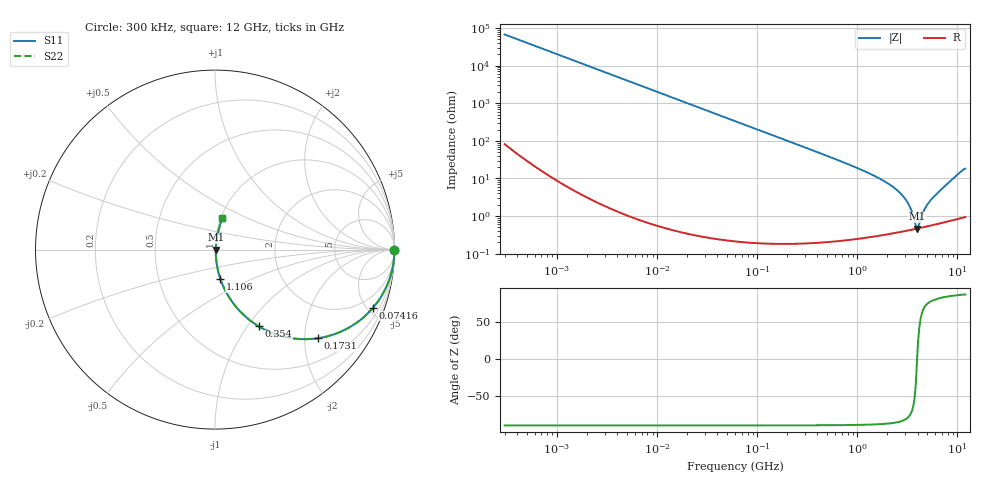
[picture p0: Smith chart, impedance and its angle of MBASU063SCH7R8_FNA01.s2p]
! MBASU063SCH7R8_FNA01  S-PARAMETER MODEL  ( General Type )
! Model Generated by TAIYO YUDEN Corporation (http://www.ty-top.com)
! Version 1.0
! TAIYO YUDEN Control No. 130801
! Copyright(c) 2013 TAIYO YUDEN CO.,LTD. All Rights Reserved.
! Product Description (link to TY-COMPAS)
! https://ds.yuden.co.jp/TYCOMPAS/or/detail?pn=MBASU063SCH7R8DFNA01&u=M
! Products Name : Multilayer Ceramic Capacitors
! Characteristics :
!  Capacitance : 7.8 pF , Rated Voltage : 50V , TCC : CH / C0H
!  Case Size : 0.6 x 0.3 / 0.024 x 0.012 [mm/inch] , Thickness : 0.3 / 0.012 [mm/inch]
!  (Conditions: Temperature = 25 degC , DC Bias Current/Voltage = 0A / 0V)
! External Node Assignments :
!  1  o---| |---o  2
! GND o---------o GND
! Frequency Range : 0.3MHz  -  12000MHz  [ 401 STEP ]
# MHz S RI R 50
! Freq[MHz].  S11 Real  S11 Imag  S21 Real  S21 Imag  S12 Real  S12 Imag  S22 Real  S22 Imag
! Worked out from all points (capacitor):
!   401 points, 300 kHz to 12 GHz, reference 50 ohm
!   read as one part in series: C = 7.88 pF near 316.3 kHz
!   lowest |Z| = 465 mohm at 3.944 GHz (marker M1)
!   series resonance near 3.949 GHz, so ESL is about 210 pH
!   S11 on the Smith chart (normalised r, x): 300 kHz: open; 74.16 MHz: 1.00, -5.45; 173.1 MHz: 1.00, -2.33; 354 MHz: 1.00, -1.13; 1.106 GHz: 1.01, -0.34; 12 GHz: 1.02, +0.37
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0.3  1 -0.00148  4.01e-06 0.00148  4.01e-06 0.00148  1 -0.00148
1.769972  0.9999 -0.00876  7.95e-05 0.00876  7.95e-05 0.00876  0.9999 -0.00876
10.44266  0.9973 -0.0515  0.00268 0.0515  0.00268 0.0515  0.9973 -0.0515
27.10171  0.9823 -0.1317  0.0177 0.1317  0.0177 0.1317  0.9823 -0.1317
60  0.9188 -0.2728  0.0812 0.2728  0.0812 0.2728  0.9188 -0.2728
74.16388  0.881 -0.3234  0.119 0.3234  0.119 0.3234  0.881 -0.3234
113.3117  0.7602 -0.4264  0.2398 0.4264  0.2398 0.4264  0.7602 -0.4264
173.124  0.5756 -0.4935  0.4244 0.4935  0.4244 0.4935  0.5756 -0.4935
353.9943  0.2435 -0.4275  0.7565 0.4275  0.7565 0.4275  0.2435 -0.4275
585.5907  0.1038 -0.3018  0.8962 0.3018  0.8962 0.3018  0.1038 -0.3018
1105.905  0.0299 -0.163  0.9701 0.163  0.9701 0.163  0.0299 -0.163
2088.533  0.00813 -0.069  0.9919 0.069  0.9919 0.069  0.00813 -0.069
2581.562  0.00568 -0.0445  0.9943 0.0445  0.9943 0.0445  0.00568 -0.0445
3026.31  0.00476 -0.0274  0.9952 0.0274  0.9952 0.0274  0.00476 -0.0274
3364.605  0.00451 -0.0164  0.9955 0.0164  0.9955 0.0164  0.00451 -0.0164
3740.715  0.00453 -0.00562  0.9955 0.00562  0.9955 0.00562  0.00453 -0.00562
3944.255  0.00463 -0.000109  0.9954 0.000109  0.9954 0.000109  0.00463 -0.000109
4158.869  0.00479 0.00431  0.9952 -0.00431  0.9952 -0.00431  0.00479 0.00431
4875.354  0.00553 0.0173  0.9945 -0.0173  0.9945 -0.0173  0.00553 0.0173
5565.855  0.00645 0.0279  0.9935 -0.0279  0.9935 -0.0279  0.00645 0.0279
9708.23  0.0215 0.1145  0.9785 -0.1145  0.9785 -0.1145  0.0215 0.1145
12000  0.0407 0.1735  0.9593 -0.1735  0.9593 -0.1735  0.0407 0.1735
